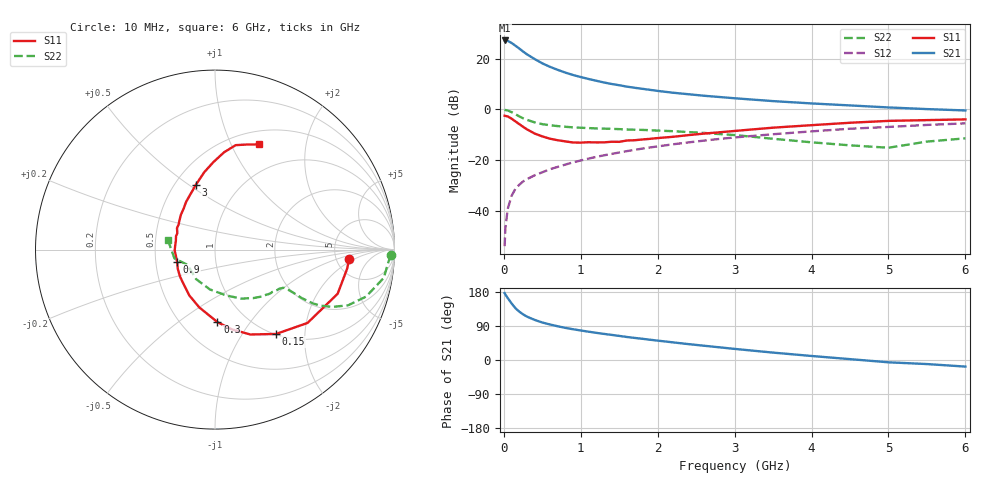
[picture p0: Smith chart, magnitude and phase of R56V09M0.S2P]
! SIEMENS Small Signal Semiconductors
! BFR183
! Si NPN RF Bipolar Junction Transistor in SOT23
! VCE = 6 V  IC = 9 mA
! Common Emitter S-Parameters:  May  1996
# GHz  S  MA  R  50
!  f  S11  S21  S12  S22
! GHz  MAG  ANG  MAG  ANG  MAG  ANG  MAG  ANG
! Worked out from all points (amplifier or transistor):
!   36 points, 10 MHz to 6 GHz, reference 50 ohm
!   highest |S21| = 27.2 dB at 10 MHz (marker M1)
!   |S21| within 3 dB of that: start of sweep to 192.1 MHz
!   unconditionally stable (mu >= 1): 835.7 MHz to 2.565 GHz
!   at 250 MHz: K = 0.58, MSG = 25.6 dB, |S12| = -28.5 dB
!   at 1.4 GHz: K = 1.05, MAG = 12.4 dB, |S12| = -17.6 dB
!   at 6 GHz: K = 0.89, MSG = 2.5 dB, |S12| = -5.5 dB
!   S11 on the Smith chart (normalised r, x): 10 MHz: 6.57, -1.61; 150 MHz: 1.01, -1.43; 300 MHz: 0.74, -0.71; 900 MHz: 0.65, -0.09; 3 GHz: 0.63, +0.53; 6 GHz: 0.65, +1.28
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0.01  0.7492 -4.1  22.9 176.5  0.002 88.6  0.9809 -1.8
0.02  0.7437 -8.3  22.78 172.9  0.0045 87.9  0.9698 -3.8
0.05  0.7263 -19.8  22.49 163.6  0.0108 79.3  0.9536 -9.5
0.1  0.6579 -38.4  20.46 149.5  0.0196 74.2  0.8814 -17.3
0.15  0.5802 -54.1  18.08 136.8  0.0271 67.7  0.8039 -22.7
0.2  0.5123 -67.4  15.89 127.7  0.0325 64.5  0.7284 -26.0
0.25  0.4535 -78.2  13.86 120.5  0.0378 62.5  0.6677 -27.9
0.3  0.404 -88.1  12.22 114.5  0.042 62.0  0.6229 -28.8
0.4  0.3338 -105.2  9.846 105.9  0.05 61.9  0.5546 -29.2
0.5  0.293 -119.1  8.097 98.9  0.0574 62.8  0.5109 -28.9
0.6  0.2639 -130.2  6.908 93.7  0.0659 63.3  0.4867 -28.8
0.7  0.246 -142.6  6.024 89.0  0.0734 64.0  0.4681 -28.7
0.9  0.222 -162.2  4.766 81.1  0.0902 64.6  0.4417 -28.9
1.1  0.2248 -178.5  3.985 74.8  0.1067 64.6  0.4277 -30.3
1.3  0.2234 167.3  3.398 68.9  0.1239 63.8  0.4168 -31.9
1.6  0.2434 150.4  2.812 60.7  0.15 62.4  0.4012 -35.4
2.2  0.2879 127.3  2.13 46.5  0.2047 58.1  0.3712 -44.5
3  0.3752 106.7  1.658 29.3  0.2794 50.0  0.3117 -61.4
3.5  0.4356 97.9  1.456 19.5  0.3233 43.9  0.263 -76.2
4.5  0.5444 84.7  1.197 2.3  0.4152 32.0  0.1952 -122.8
5.5  0.6138 72.6  1.013 -10.7  0.4932 20.2  0.2314 -167.7
6  0.635 67.3  0.952 -17.4  0.5298 12.6  0.2683 168.2
